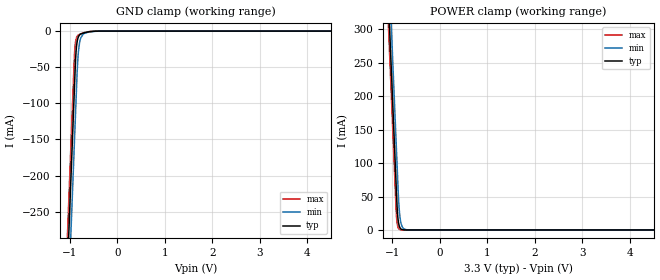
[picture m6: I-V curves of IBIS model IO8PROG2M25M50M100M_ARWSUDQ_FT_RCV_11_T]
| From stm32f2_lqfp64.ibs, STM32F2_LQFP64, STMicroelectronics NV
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| *** New cell (Generated with 5.14beta1 (Sep 20 2010 13:23:23))
[Model]   IO8PROG2M25M50M100M_ARWSUDQ_FT_RCV_11_T
Model_type Input
Polarity   Non-Inverting
Enable   Active-Low
| CAP_THRESHOLD on pad IOV33 is "CMOS" :
| Rising=10.0% of vddio   Falling=90.0% of vddio
| C_comp min and max val. don't necessarily correlate with the min and max pvt
| but are the smallest and greatest pad capacitance found.
| var   typ   min   max
C_comp   2.33710pF  2.22150pF  2.46630pF
Vinl = 800.0mV | Dummy value overriden by next lines
Vinh = 2.00V | Dummy value overriden by next lines
[Model Spec]
| TIME_THRESHOLD on pin ZIV33 is "CORE" :
| Rising=40.0% of vddio   Falling=60.0% of vddio
Vinl 1.48450V 1.23350V 1.61250V
Vinh 1.48450V 1.23350V 1.61250V
| variable   typ   min   max
[Temperature Range] 25.0 125.0 -40.0
| variable   typ   min   max
[Voltage Range] 3.3V 2.7V 3.6V
| variable   typ   min   max
[POWER Clamp Reference] 3.3V 2.7V 3.6V
| variable   typ   min   max
[GND Clamp Reference] 0V 0V 0V
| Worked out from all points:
|   GND clamp passes 1 mA (typ) near -0.61 V on its own axis
|   POWER clamp passes 1 mA (typ) near -0.81 V on its own axis
[POWER Clamp]
-3.3V     4.11A      4.173A     4.072A
-1.09V    352.5mA    415.9mA    314.5mA
-1.05V    284.5mA    347.9mA    246.5mA
-1.01V    216.5mA    279.9mA    178.5mA
-920mV    63.51mA    126.9mA    25.85mA
-900mV    31.51mA    92.9mA     9.552mA
-890mV    21.35mA    75.9mA     5.807mA
-870mV    9.804mA    44.01mA    2.146mA
-840mV    3.05mA     18.36mA    482.1uA
-780mV    295.2uA    3.194mA    24.34uA
-660mV    2.764uA    96.52uA    62.42nA
6.6V      0A         0A         0A
[GND Clamp]
-3.3V     -4.149A    -4.224A    -4.103A
-1.06V    -341mA     -415.8mA   -295.1mA
-940mV    -137mA     -211.8mA   -91.11mA
-900mV    -69.01mA   -143.8mA   -27.13mA
-880mV    -37.2mA    -109.8mA   -14.07mA
-870mV    -27.03mA   -92.82mA   -10.89mA
-840mV    -11.77mA   -45.3mA    -6.542mA
-810mV    -6.468mA   -21.54mA   -4.94mA
-780mV    -4.366mA   -11.11mA   -3.995mA
-700mV    -2.247mA   -3.206mA   -2.168mA
-350mV    -8.284uA   -44.58uA   -1.618uA
6.6V      10.47nA    1.304uA    84.25pA
